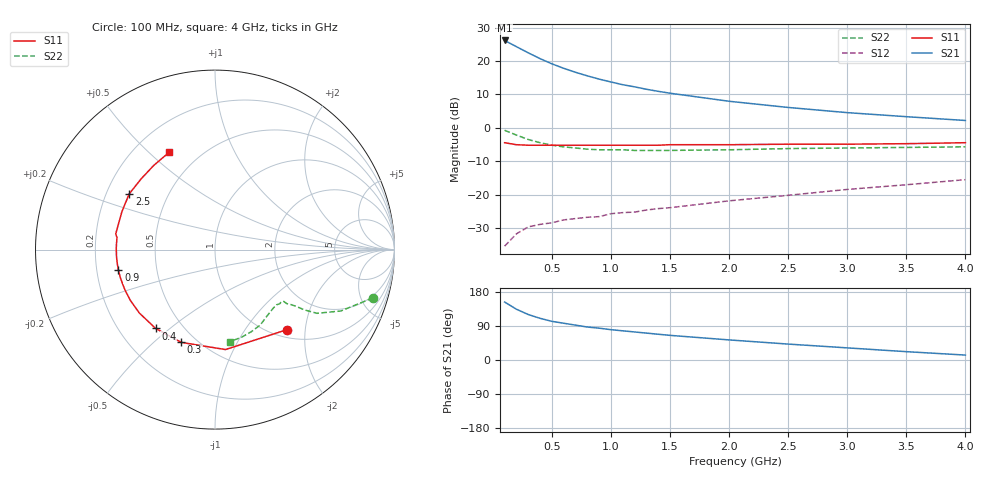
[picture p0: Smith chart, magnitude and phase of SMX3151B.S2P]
! HSMX-3151 COMMON EMITTER
! Vce=10V Ic=10ma
# ghz s ma r 50
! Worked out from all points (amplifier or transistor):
!   20 points, 100 MHz to 4 GHz, reference 50 ohm
!   highest |S21| = 26.1 dB at 100 MHz (marker M1)
!   |S21| within 3 dB of that: start of sweep to 262 MHz
!   unconditionally stable (mu >= 1): 1.076 GHz to 3.626 GHz
!   at 400 MHz: K = 0.52, MSG = 24.8 dB, |S12| = -28.9 dB
!   at 1.1 GHz: K = 1.01, MAG = 18.4 dB, |S12| = -25.4 dB
!   at 4 GHz: K = 0.93, MSG = 8.9 dB, |S12| = -15.5 dB
!   lowest NFmin = 1.90 dB at 500 MHz
!   S11 on the Smith chart (normalised r, x): 100 MHz: 1.15, -1.60; 300 MHz: 0.42, -0.62; 400 MHz: 0.36, -0.45; 900 MHz: 0.29, -0.10; 2.5 GHz: 0.30, +0.27; 4 GHz: 0.34, +0.58
0.1  0.6 -48.0  20.3 153.0  0.017 68.0  0.92 -17.0
0.2  0.56 -84.0  16.39 134.0  0.026 56.0  0.78 -26.0
0.3  0.55 -110.0  13.26 120.0  0.033 50.0  0.67 -32.0
0.4  0.55 -127.0  10.86 110.0  0.036 47.0  0.6 -34.0
0.5  0.55 -140.0  9.08 102.0  0.038 46.0  0.55 -35.0
0.6  0.55 -149.0  7.78 97.0  0.042 45.0  0.52 -36.0
0.7  0.55 -156.0  6.78 92.0  0.044 46.0  0.5 -37.0
0.8  0.55 -163.0  6 87.0  0.046 48.0  0.48 -37.0
0.9  0.55 -168.0  5.36 84.0  0.047 47.0  0.47 -38.0
1  0.55 -172.0  4.86 80.0  0.052 49.0  0.47 -39.0
1.1  0.55 -176.0  4.42 77.0  0.054 48.0  0.47 -40.0
1.2  0.55 -180.0  4.11 74.0  0.055 52.0  0.46 -42.0
1.3  0.55 177.0  3.78 71.0  0.059 53.0  0.46 -43.0
1.4  0.55 173.0  3.52 68.0  0.062 53.0  0.46 -44.0
1.5  0.56 171.0  3.3 65.0  0.064 55.0  0.46 -45.0
2  0.56 158.0  2.5 53.0  0.081 58.0  0.47 -52.0
2.5  0.57 147.0  2.02 42.0  0.098 60.0  0.49 -59.0
3  0.57 136.0  1.69 32.0  0.12 58.0  0.5 -66.0
3.5  0.58 126.0  1.47 22.0  0.141 58.0  0.51 -73.0
4  0.6 115.0  1.29 13.0  0.168 56.0  0.52 -81.0
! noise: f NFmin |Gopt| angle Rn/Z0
0.5  1.9  0.07  91  0.38
1  2  0.23  127  0.18
1.5  2.3  0.39  145  0.1
2  2.5  0.36  180  0.2
